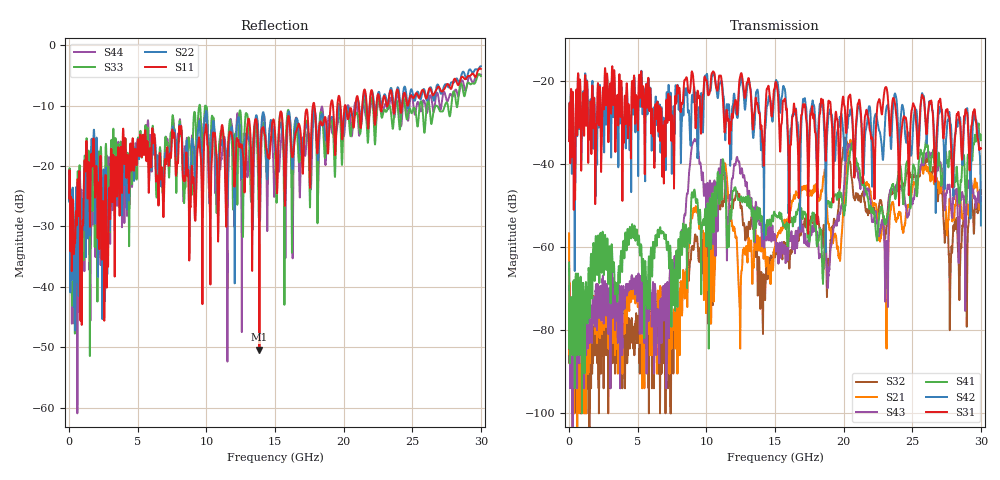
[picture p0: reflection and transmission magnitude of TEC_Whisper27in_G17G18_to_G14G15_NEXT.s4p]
! Tyco Electronics
! G17G18-G14G15_NEXT
!! PART DESCRIPTION: Whisper 27in Megtron 6 VLP-HVLP-VLP Channel Model, bulkhead 2.4mm test pts
!! MODEL DESCRIPTION: System 4-port S-parameter
!! MODEL STATUS: Measured
!! MODEL GEOMETRY: Channel Model
!! MODEL FREQUENCY RANGE: DC to 30.000 GHz in 10.000 MHz frequency steps
!! MODEL EDGE RATE LIMITATION: 12.500 ps (Using conservative 0.5/Fmax rule of thumb)
!! TIME-DOMAIN TRANSFORM CAUTIONS:
!! 1.) Do not simulate transient edge rates faster than the number listed above.  Edge rates faster than this number
!!  contain significant spectral content at frequencies above the model's highest frequency.
!! 2.) Even when simulating edge rates that are slower than the number listed above, be aware that the best time
!!  resolution possible with a direct iFFT is (1 / 2Fmax).  As a result, time resolution is typically not adequate
!!  for most time-domain simulations unless tricks such as windowing are used to minimize leakage and aliasing.
!! 3.) Because the model has a uniform frequency step, a direct iFFT will result in an impulse that that has a time
!!  length given by either (1 / Fstep) or (1 / 2Fstep), depending on the transform being used.  Care has been taken
!!  in selecting the frequency step to ensure a settled impulse response for the model.  Therefore, convolution with
!!  the model's impulse response should present no issues.  However, if directly concatenating s-parameter models
!!  in the frequency domain a user must either interpolate necessary interim frequencies or complete impulse response
!!  zero-padding.  Impulse response zero-padding is more difficult, but more accurate.
!! PORT DEFINITIONS:
!! Port  1  ----->  Side A  G17  G14  Side A  <-----  Port  2
!! Port  3  ----->  Side A  G18  G15  Side A  <-----  Port  4
! Point-to-Point link (differential)  !
! Connectors:  !
!  1: STRADA Whisper  !
! Materials:  !
!  Backplane: Megtron-6 HVLP  !
!  Daughtercard: Megtron-6 VLP  !
! Stack-up:  !
!  Backplane: 20 layers, 200mil thick  !
!  Daughtercard: 14 layers, 110mil thick  !
! Trace Length:  !
!  Backplane: 17in  !
!  Daightercards: 5in  !
! Trace Width:  !
!  Backplane: 8-13-8 mils  !
!  Daughtercards: 6-9-6 mils  !
! Geometry:  !
!  Backplane: Stripline  !
!  Daughtercards: Stripline  !
! Freq. Range: 0 GHz - 30 GHz  !
! Note1: non-mixed-mode s-parameters  !
! Note2: channel includes 2.4mm test points  !
! Touchstone data converted from IdEM dataset
# GHz S MA R 50
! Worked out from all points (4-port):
!   3000 points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, 10 MHz to 30 GHz, reference 50 ohm
!   strongest paths, dB at 10 MHz, 7.51 GHz, 15.01 GHz, 22.51 GHz, 30 GHz:
!     S31: -34.5, -28.3, -21.1, -25.2, -36.3
!     S42: -34.5, -34.3, -21.3, -30.6, -54.8
!     S41: -63.7, -63.9, -52.1, -55.7, -34.3
!     S43: -69.6, -64.6, -57.1, -55.8, -49.0
!     S21: -56.7, -80.0, -59.8, -54.6, -51.3
!     S32: -65.2, -80.9, -62.5, -51.4, -47.3
!   lowest |S11| = -50.4 dB at 13.87 GHz (marker M1), VSWR 1.01, Z = 49.7 - j0.167 ohm
!   |S11| at or under -10 dB: start of sweep to 17.77 GHz; 17.88 GHz to 19.06 GHz (1.179 GHz wide, 6.38 % of centre); 20.14 GHz to 20.87 GHz (726.3 MHz wide, 3.54 % of centre)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
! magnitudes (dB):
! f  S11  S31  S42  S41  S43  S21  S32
! 10 MHz  -25.4  -34.5  -34.5  -63.7  -69.6  -56.7  -65.2
! 6.48 GHz  -22.9  -27.4  -25.4  -56.0  -75.4  -71.7  -88.0
! 9.15 GHz  -28.2  -24.6  -23.0  -46.3  -34.0  -51.6  -58.0
! 13.87 GHz  -50.4  -27.7  -27.4  -50.7  -54.5  -59.5  -64.3
! 18.88 GHz  -17.7  -25.3  -29.0  -48.9  -68.2  -54.3  -63.1
! 20.12 GHz  -9.9  -28.3  -36.5  -50.0  -40.2  -43.9  -33.7
! 30 GHz  -4.0  -36.3  -54.8  -34.3  -49.0  -51.3  -47.3
